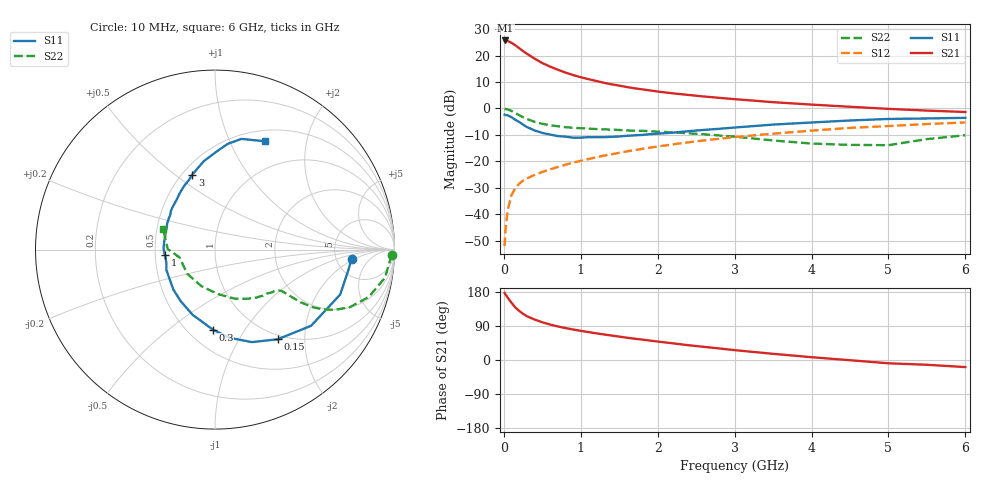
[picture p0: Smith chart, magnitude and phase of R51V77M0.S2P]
! SIEMENS Small Signal Semiconductors
! BFR183
! Si NPN RF Bipolar Junction Transistor in SOT23
! VCE = 1.75 V  IC = 7 mA
! Common Emitter S-Parameters:  May  1996
# GHz  S  MA  R  50
!  f  S11  S21  S12  S22
! GHz  MAG  ANG  MAG  ANG  MAG  ANG  MAG  ANG
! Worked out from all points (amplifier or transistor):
!   36 points, 10 MHz to 6 GHz, reference 50 ohm
!   highest |S21| = 25.7 dB at 20 MHz (marker M1)
!   |S21| within 3 dB of that: start of sweep to 203.8 MHz
!   unconditionally stable (mu >= 1): 856.6 MHz to 2.597 GHz
!   at 250 MHz: K = 0.52, MSG = 24.5 dB, |S12| = -27.3 dB
!   at 1.4 GHz: K = 1.07, MAG = 11.7 dB, |S12| = -17.3 dB
!   at 6 GHz: K = 0.90, MSG = 2.0 dB, |S12| = -5.3 dB
!   S11 on the Smith chart (normalised r, x): 10 MHz: 6.96, -1.77; 150 MHz: 0.93, -1.48; 300 MHz: 0.66, -0.73; 1 GHz: 0.56, -0.04; 3 GHz: 0.56, +0.58; 6 GHz: 0.63, +1.37
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0.01  0.7624 -4.0  19.09 177.1  0.0025 87.1  0.9863 -1.8
0.02  0.7525 -8.4  19.29 173.6  0.005 84.9  0.9761 -3.8
0.05  0.7409 -19.8  18.87 164.6  0.0121 80.3  0.96 -9.4
0.1  0.6832 -38.4  17.38 151.0  0.0231 72.6  0.8966 -17.1
0.15  0.6094 -55.1  15.62 138.5  0.0313 66.3  0.817 -23.1
0.2  0.5548 -68.3  13.79 129.5  0.0379 62.6  0.7457 -26.8
0.25  0.4973 -80.8  12.14 121.9  0.0433 60.0  0.6838 -29.1
0.3  0.4455 -91.6  10.81 115.5  0.0478 59.0  0.633 -30.5
0.4  0.3843 -108.9  8.741 106.8  0.0555 58.3  0.5592 -31.6
0.5  0.3447 -123.8  7.212 99.5  0.0632 58.5  0.5131 -31.7
0.6  0.3218 -136.1  6.189 93.7  0.0706 59.2  0.4829 -31.7
0.8  0.2936 -157.3  4.772 84.3  0.0865 60.4  0.4435 -31.8
1  0.281 -173.7  3.893 77.0  0.1025 61.1  0.4239 -32.6
1.1  0.2869 179.0  3.584 73.7  0.1109 61.3  0.4156 -33.6
1.3  0.2868 166.5  3.063 67.4  0.1284 61.1  0.4027 -35.2
1.6  0.3044 150.9  2.54 58.8  0.1544 60.3  0.3851 -39.0
2.2  0.3495 128.0  1.929 43.9  0.2102 56.6  0.354 -48.9
3  0.4362 106.9  1.5 26.0  0.2881 48.6  0.2936 -68.3
3.5  0.4962 97.3  1.315 16.3  0.3341 42.6  0.2487 -86.1
4.5  0.5929 83.2  1.077 -0.6  0.4295 30.2  0.2052 -138.7
5.5  0.6473 70.3  0.912 -12.6  0.5078 18.0  0.2636 179.3
6  0.6657 65.0  0.858 -18.7  0.5442 10.1  0.312 158.0
